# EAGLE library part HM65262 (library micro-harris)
MICROCONTROLLER/MEMORY DEVICE
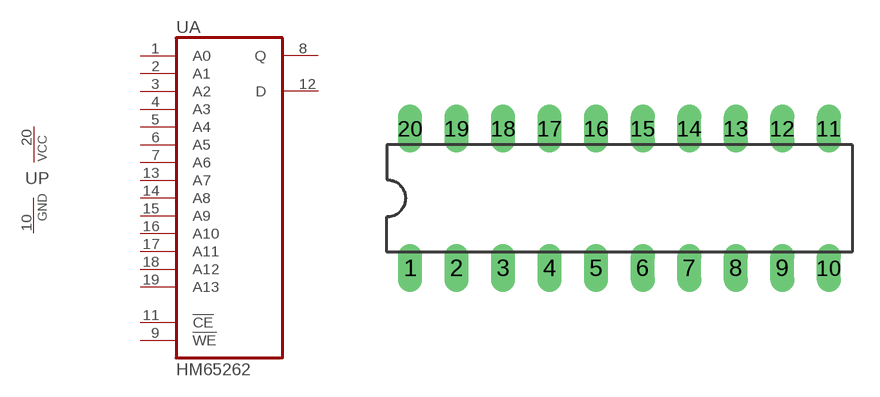
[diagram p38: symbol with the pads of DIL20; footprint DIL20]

Designator prefix U; gates A=HM65262 P=PWRN

## HM65262 (OC_FARNELL: unknown; OC_NEWARK: unknown)  [DIL20]
1  A:A0  in
2  A:A1  in
3  A:A2  in
4  A:A3  in
5  A:A4  in
6  A:A5  in
7  A:A6  in
8  A:Q  hiz
9  A:!WE  in
10  P:GND  pwr
11  A:!CE  in
12  A:D  in
13  A:A7  in
14  A:A8  in
15  A:A9  in
16  A:A10  in
17  A:A11  in
18  A:A12  in
19  A:A13  in
20  P:VCC  pwr

## Footprint DIL20 (pad centres in mm)
Dual In Line Package
drill 0.813 long: 1 -11.43,-3.81; 2 -8.89,-3.81; 3 -6.35,-3.81; 4 -3.81,-3.81; 5 -1.27,-3.81; 6 1.27,-3.81; 7 3.81,-3.81; 8 6.35,-3.81; 9 8.89,-3.81; 10 11.43,-3.81; 11 11.43,3.81; 12 8.89,3.81; 13 6.35,3.81; 14 3.81,3.81; 15 1.27,3.81; 16 -1.27,3.81; 17 -3.81,3.81; 18 -6.35,3.81; 19 -8.89,3.81; 20 -11.43,3.81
